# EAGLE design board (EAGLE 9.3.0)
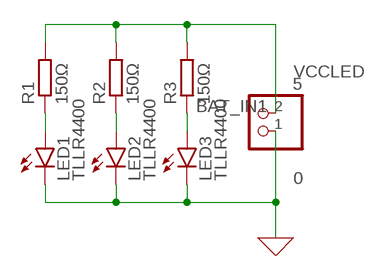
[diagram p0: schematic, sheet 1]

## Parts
BAT_IN1  5  PINHD-1X2  [1X02]
LED1  TLLR4400  [LED3MM]
LED2  TLLR4400  [LED3MM]
LED3  TLLR4400  [LED3MM]
R1  150Ω  R-EU_0204/7  [0204/7]
R2  150Ω  R-EU_0204/7  [0204/7]
R3  150Ω  R-EU_0204/7  [0204/7]

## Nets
0: BAT_IN1.1 LED1.K(C) LED2.K(C) LED3.K(C) ; supply symbol labelled GND
N$5: LED1.A R1.1
N$11: LED2.A R2.1
N$12: LED3.A R3.1
VCCLED: BAT_IN1.2 R1.2 R2.2 R3.2

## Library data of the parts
BAT_IN1 = pinhead:PINHD-1X2: PIN HEADER; SPICEPREFIX: V
LED1-LED3 = led:TLLR4400: Low Current (2mA) LED 3 mm Tinted Diffused Package color RED; MF: VISHAY SEMICONDUCTOR; OC_FARNELL: 1612437; SPICEMODEL: DMOD; SPICEPREFIX: D
R1-R3 = rcl:R-EU_: RESISTOR, European symbol; SPICEPREFIX: R

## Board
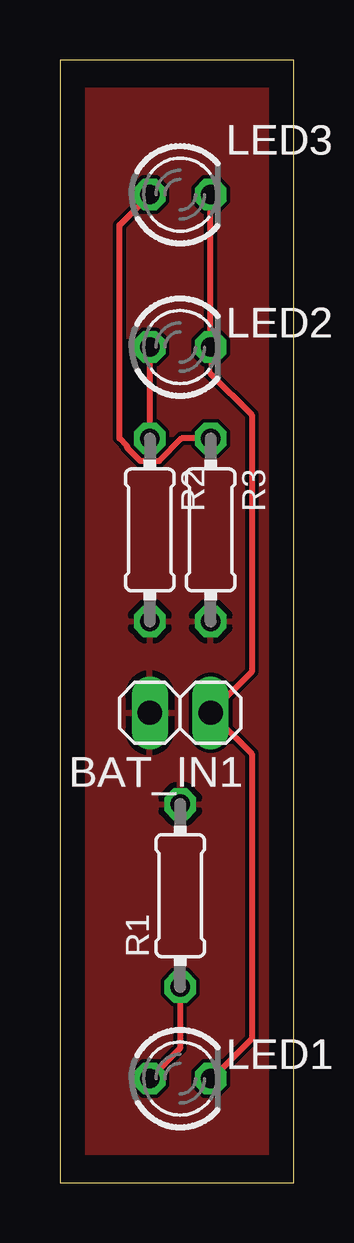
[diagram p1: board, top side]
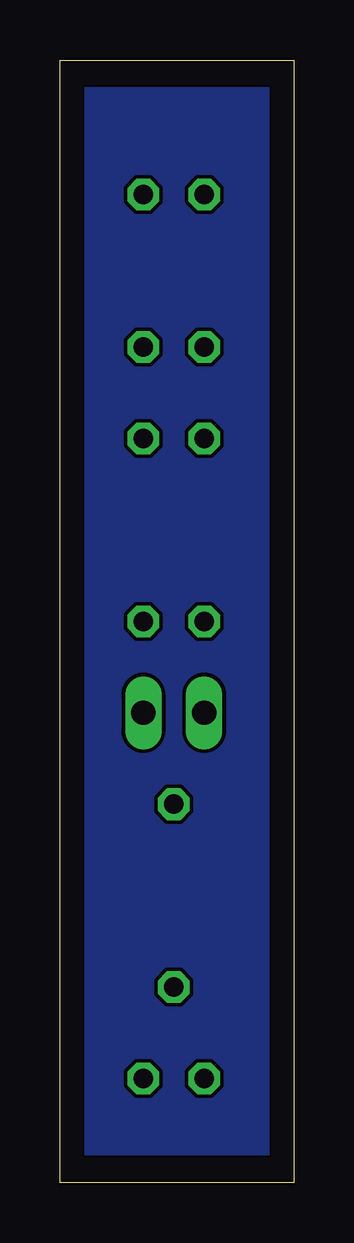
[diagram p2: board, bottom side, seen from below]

Size 9.77 x 46.79 mm. Coordinates in mm from the lower left corner, seen from the top.
Outline: 0,0 9.77,0 9.77,46.79 0,46.79 0,0
Copper layers (1*16): Top 0.035mm / dielectric 1.5mm / Bottom 0.035mm
Design rules "default *": minimum track width 6mil, minimum drill 0.35mm, track to track 6mil, track to pad 6mil, pad to pad 6mil, via to via 6mil, smd to smd 6mil, copper to edge 40mil, drill to drill 6mil, minimum pad ring 10mil, minimum via ring 8mil, stop-mask expansion 4mil, vias tented up to drill 0mil, thermal gap 10mil

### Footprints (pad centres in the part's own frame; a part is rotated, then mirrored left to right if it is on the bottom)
1X02 = drill 1.016 long: 1 -1.27,0; 2 1.27,0
LED3MM = drill 0.813 octagon: A -1.27,0; K 1.27,0
0204/7 = drill 0.813 octagon: 1 -3.81,0; 2 3.81,0

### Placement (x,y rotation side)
BAT_IN1  5.02,19.59 180 top
LED1  5.02,4.35 0 top
LED2  5.02,34.83 0 top
LED3  5.02,41.18 0 top
R1  5.02,11.97 90 top
R2  3.75,27.21 270 top
R3  6.29,27.21 270 top

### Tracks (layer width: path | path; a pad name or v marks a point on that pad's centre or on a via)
0
  Top 0.152: LED2.K 6.29,33.71 | 6.35,4.35 LED1.K
  Top 0.254: 6.29,33.71 8,32 8,21.3 BAT_IN1.1 8,17.88 8,6 6.35,4.35 | LED2.K LED3.K
GNDLED
  pour Bottom: 0.94,45.53 8.83,45.53 8.83,1.27 0.94,1.27
N$5
  Top 0.254: R1.1 5.02,5.62 LED1.A
N$11
  Top 0.254: R2.1 LED2.A
N$12
  Top 0.254: R3.1 5.08,31.02 4.14,30.08 3.36,30.08 2.81,30.63 2.81,30.69 2.48,31.02 2.48,39.91 LED3.A
VCCLED
  pour Top: 0.94,45.53 8.83,45.53 8.83,1.27 0.94,1.27

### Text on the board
_tNames: LED3 | LED2 | R2 | R3 | BAT_IN1 | R1 | LED1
